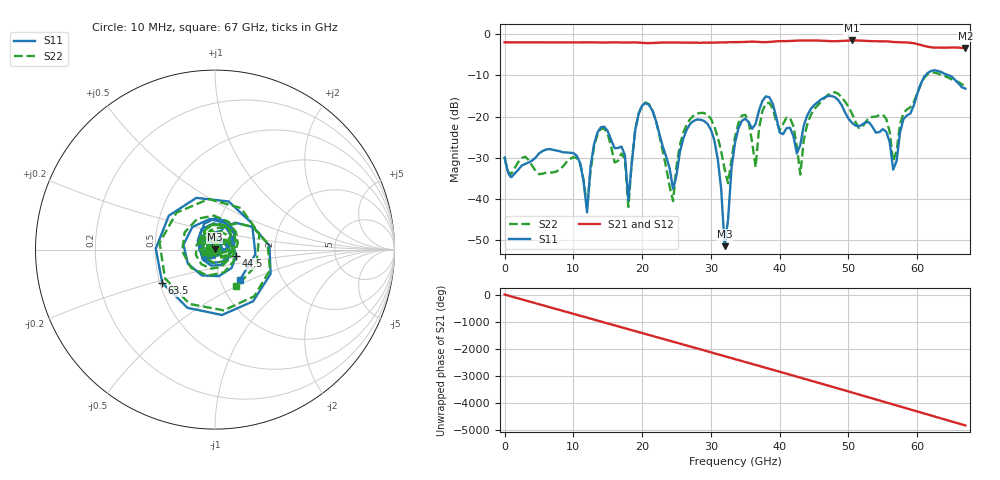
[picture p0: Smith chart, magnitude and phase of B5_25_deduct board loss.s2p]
!Keysight Technologies,N5247B,MY61255065,A.16.20.04
!Date: Monday, September 04, 2023 01:14:40
!Correction: S11(C  2-Port  )
!S21(C  2-Port  )
!S12(C  2-Port  )
!S22(C  2-Port  )
!S2P File: Measurements: S11, S21, S12, S22:
!Deduct Board Loss
# Hz S  dB  R 50
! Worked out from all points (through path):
!   142 points, 10 MHz to 67 GHz, reference 50 ohm
!   highest |S21| = -1.50 dB at 50.5 GHz (marker M1); lowest = -3.3 dB at 67 GHz (marker M2)
!   lowest |S11| = -51.5 dB at 32 GHz (marker M3), VSWR 1.01, Z = 49.9 + j0.248 ohm
!   |S11| at or under -10 dB: start of sweep to 61.18 GHz; 64.62 GHz to end of sweep
!   |S22| runs from -42.2 to -9.3 dB; largest |S21 - S12| = 0.0039
!   S11 on the Smith chart (normalised r, x): 10 MHz: 0.94, -0.00; 44.5 GHz: 1.26, -0.09; 63.5 GHz: 0.51, -0.22; 67 GHz: 1.23, -0.44
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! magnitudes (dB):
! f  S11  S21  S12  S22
! 10 MHz  -29.9  -2.0  -2.0  -29.9
! 11.5 GHz  -35.8  -2.0  -2.0  -35.4
! 12 GHz  -43.3  -2.0  -2.0  -42.2
! 14.5 GHz  -22.5  -2.0  -2.0  -22.9
! 18 GHz  -40.3  -2.0  -2.0  -41.9
! 20 GHz  -17.3  -2.1  -2.1  -17.2
! 22.5 GHz  -24.1  -2.0  -2.0  -24.4
! 24.5 GHz  -37.5  -2.0  -2.0  -40.5
! 26.5 GHz  -23.1  -2.0  -2.0  -21.9
! 30 GHz  -23.2  -2.0  -2.0  -20.5
! 32 GHz  -51.5  -1.9  -1.9  -32.8
! 34 GHz  -22.9  -1.9  -1.9  -21.6
! 36.5 GHz  -21.8  -1.8  -1.8  -32.3
! 38 GHz  -15.1  -1.9  -1.9  -16.8
! 41.5 GHz  -22.7  -1.6  -1.6  -20.3
! 43 GHz  -26.9  -1.5  -1.5  -34.1
! 44.5 GHz  -18.2  -1.5  -1.5  -19.7
! 45 GHz  -17.2  -1.5  -1.5  -18.2
! 50.5 GHz  -21.5  -1.5  -1.5  -19.2
! 56 GHz  -26.2  -1.8  -1.8  -23.7
! 63.5 GHz  -9.2  -3.3  -3.3  -9.9
! 67 GHz  -13.2  -3.3  -3.4  -12.5
